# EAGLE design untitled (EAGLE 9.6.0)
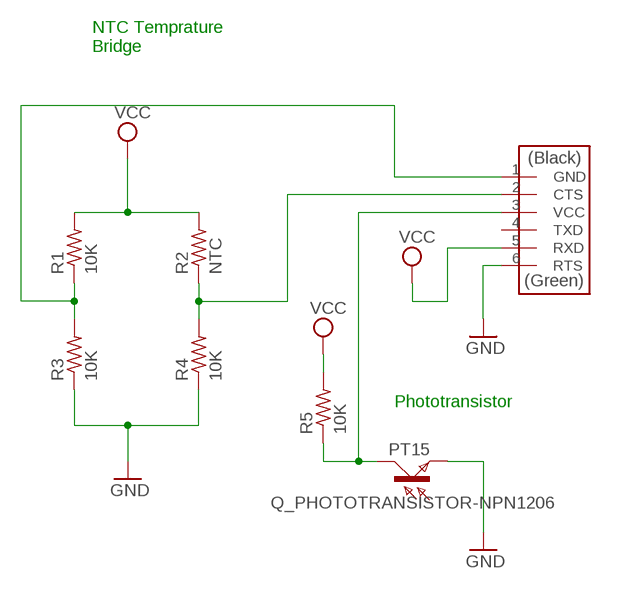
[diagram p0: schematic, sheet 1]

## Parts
PT15  Q_PHOTOTRANSISTOR-NPN1206  [OP1206]
R1  10K  R1206FAB  [R1206FAB]
R2  NTC  R1206FAB  [R1206FAB]
R3  10K  R1206FAB  [R1206FAB]
R4  10K  R1206FAB  [R1206FAB]
R5  10K  R1206FAB  [R1206FAB]
U$1  CONN_06_FTDI-SMD-HEADER  [1X06SMD]

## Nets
GND: PT15.EMITTER(E) R3.1 R4.1 U$1.6(RTS)
N$1: R1.1 R3.2 U$1.1(GND)
N$2: PT15.COLLECTOR(C) R5.1 U$1.3(VCC)
N$4: R2.1 R4.2 U$1.2(CTS)
VCC: R1.2 R2.2 R5.2 U$1.5(RXD)
Unconnected: U$1.4(TXD)

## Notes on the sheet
- NTC Temprature
  Bridge
- Phototransistor

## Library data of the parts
PT15 = fab:Q_PHOTOTRANSISTOR-NPN
R1-R5 = fab:R: Resistor (US Symbol)
U$1 = fab:CONN_06_FTDI-SMD-HEADER

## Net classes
0 default: width 0.406 mm

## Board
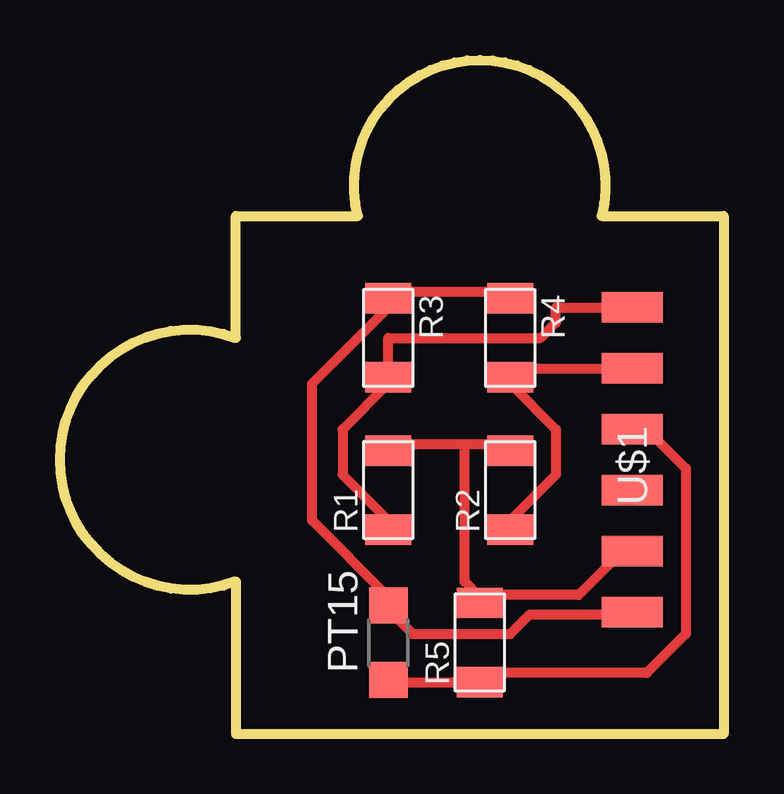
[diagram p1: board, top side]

Size 27.65 x 28.1 mm. Coordinates in mm from the lower left corner, seen from the top.
Outline: 12.41,21.59 arc-208 22.57,21.59 27.65,21.59 27.65,0 7.33,0 7.33,6.35 arc-221 7.33,16.51 7.33,21.59 12.41,21.59
Copper layers (1*16): Top 0.035mm / dielectric 1.5mm / Bottom 0.035mm
Design rules "fab": minimum track width 10mil, minimum drill 32mil, track to track 16mil, track to pad 16mil, pad to pad 16mil, via to via 16mil, smd to smd 6mil, copper to edge 16mil, drill to drill 16mil, minimum pad ring 10mil, minimum via ring 8mil, stop-mask expansion 4mil, vias tented up to drill 0mil, thermal gap 16mil

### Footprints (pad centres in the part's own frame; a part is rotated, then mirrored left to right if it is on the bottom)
OP1206 = smd 1.5 x 1.6: COLLECTOR -1.55,0; EMITTER 1.55,0
R1206FAB = smd 1.27 x 1.905: 1 -1.651,0; 2 1.651,0
1X06SMD = smd 2.54 x 1.27: 1 0,6.35; 2 0,3.81; 3 0,1.27; 4 0,-1.27; 5 0,-3.81; 6 0,-6.35

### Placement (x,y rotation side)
PT15  13.68,3.81 90 top
R1  13.68,10.16 90 top
R2  18.76,10.16 90 top
R3  13.68,16.51 270 top
R4  18.76,16.51 270 top
R5  17.49,3.81 90 top
U$1  23.84,11.43 0 top

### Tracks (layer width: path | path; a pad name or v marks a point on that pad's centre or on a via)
GND
  Top 0.406: 13.68,5.08 PT15.EMITTER | U$1.6 23.64,4.98 19.57,4.98 18.76,4.17 14.7,4.17 13.88,4.98 PT15.EMITTER | R4.1 18.76,18.41 13.68,18.41 R3.1 13.68,17.78 10.51,14.61 10.51,8.89 13.68,5.72 PT15.EMITTER
N$1
  Top 0.406: R1.1 13.68,8.89 11.78,10.79 11.78,12.7 13.68,14.61 R3.2 13.68,16.51 20.03,16.51 20.67,17.14 20.67,17.78 U$1.1
N$2
  Top 0.406: 24.45,12.7 24.48,12.7 | 13.68,2.54 PT15.COLLECTOR 13.88,2.13 17.13,2.13 R5.1 | 17.49,2.54 R5.1 | 24.45,12.7 26.08,11.07 26.08,4.17 24.45,2.54 17.54,2.54 R5.1 | 24.45,12.7 U$1.3
N$4
  Top 0.406: 18.56,14.73 R4.2 | R2.1 18.76,8.89 20.67,10.79 20.67,12.7 18.76,14.61 R4.2 | U$1.2 18.76,15.24 R4.2
VCC
  Top 0.406: R5.2 17.54,5.79 21.61,5.79 23.64,7.82 U$1.5 | 17.13,5.79 R5.2 | 16.86,12.06 18.76,12.06 R2.2 | 16.86,12.06 13.68,12.06 R1.2 | 16.86,12.06 16.86,6.35 17.49,5.72 R5.2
